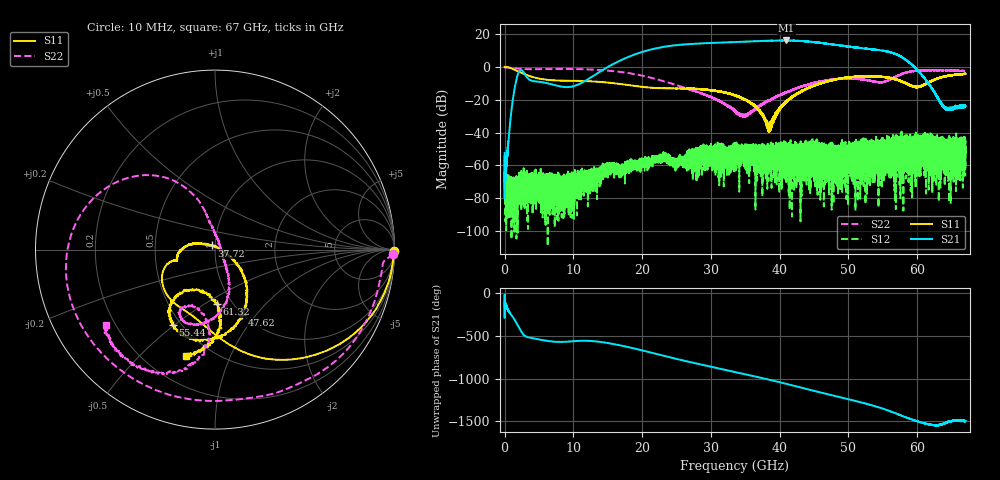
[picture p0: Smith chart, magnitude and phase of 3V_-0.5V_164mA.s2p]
! MARKI MICROWAVE INC.
! Date:  10/21/2020
! Model Number:  AMM-7210CH
! Description:  2-port Small Signal S-parameter data for AMM-7210CH
! Frequency Range:  10 MHz to 67 GHz
! Port Configuration:  PORT 1: Input
!  PORT 2: Output
! Bias Condition: Vd = +3.0V, Vg = -0.5V
! AMM-7210CH s2p files are only valid for small signal conditions (below -10 dBm input power)
# Hz S  dB  R 50
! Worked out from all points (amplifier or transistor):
!   20001 points, 10 MHz to 67 GHz, reference 50 ohm
!   highest |S21| = 16.0 dB at 40.96 GHz (marker M1)
!   |S21| within 3 dB of that: 24.7 GHz to 48.71 GHz (24 GHz wide, 65.4 % of centre)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
!   unconditionally stable (mu >= 1): start of sweep to end of sweep
!   at 11.17 GHz: K = 991.82, MAG = -3.8 dB, |S12| = -68.2 dB
!   at 33.51 GHz: K = 44.51, MAG = 15.1 dB, |S12| = -54.2 dB
!   at 67 GHz: K = 4730.73, MAG = -18.4 dB, |S12| = -66.6 dB
!   S11 on the Smith chart (normalised r, x): 10 MHz: open; 37.72 GHz: 0.96, +0.04; 47.62 GHz: 0.99, -0.85; 55.44 GHz: 0.45, -0.49; 61.32 GHz: 0.85, -0.57; 67 GHz: 0.38, -0.69
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1e7  -0.04 -0.4  -52.34 -147.6  -55.17 -176.2  -0.06 -1.5
2.230718e9  -3.25 -62.6  -2.30 -62.7  -75.41 -174.8  -1.17 -61.7
1.117723e10  -8.62 -133.0  -9.85 161.8  -68.79 -177.4  -1.48 -168.8
1.700201e10  -10.56 -160.6  4.14 105.4  -61.16 149.0  -3.23 149.4
1.989263e10  -12.13 -165.0  8.86 52.2  -56.87 116.6  -5.27 130.5
2.234112e10  -12.98 -164.0  11.49 3.4  -55.99 96.0  -7.82 117.5
2.470921e10  -13.22 -164.5  13.01 -43.7  -57.33 95.7  -10.72 108.5
2.774051e10  -13.38 -170.8  14.04 -101.2  -54.67 58.4  -14.95 101.8
3.087899e10  -14.74 178.7  14.61 -157.3  -53.68 3.4  -20.24 91.4
3.3505e10  -17.35 166.4  15.04 156.8  -54.21 25.0  -27.18 63.4
3.771532e10  -30.56 129.6  15.72 81.7  -55.41 -75.8  -22.04 -49.1
4.096099e10  -21.70 -24.0  16.00 19.7  -51.21 -99.4  -15.73 -62.5
4.269603e10  -16.04 -32.9  15.75 -15.4  -57.62 135.6  -12.66 -70.0
4.467223e10  -12.07 -47.2  15.18 -55.7  -50.70 96.1  -10.20 -79.7
4.761979e10  -8.11 -67.4  13.64 -114.3  -54.23 123.3  -7.71 -96.9
5.119706e10  -6.07 -92.0  11.66 175.5  -50.63 -110.2  -7.37 -116.0
5.357855e10  -5.86 -108.0  10.53 124.9  -48.17 162.1  -8.88 -118.4
5.544422e10  -6.36 -119.4  9.48 77.3  -48.13 -156.4  -8.82 -100.7
5.583612e10  -6.57 -121.7  9.11 66.5  -59.66 -160.3  -8.19 -97.5
5.86162e10  -10.63 -127.8  3.33 -19.3  -51.27 156.1  -3.26 -104.3
6.13226e10  -10.31 -87.7  -8.36 -86.7  -53.12 69.4  -2.11 -123.0
6.7e10  -4.43 -105.4  -23.90 -53.7  -66.61 11.8  -2.53 -145.4
